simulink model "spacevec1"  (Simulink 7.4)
settings: Solver=ode45  StartTime=0.0  StopTime=.02  MaxStep=.00333  RelTol=1e-4
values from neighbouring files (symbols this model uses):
  j = sqrt(-1)    [im3d.m]    (also in imbar1.m; imbarB.m; imchplot66.m; imdef0vec.m)
libraries: simulink x2

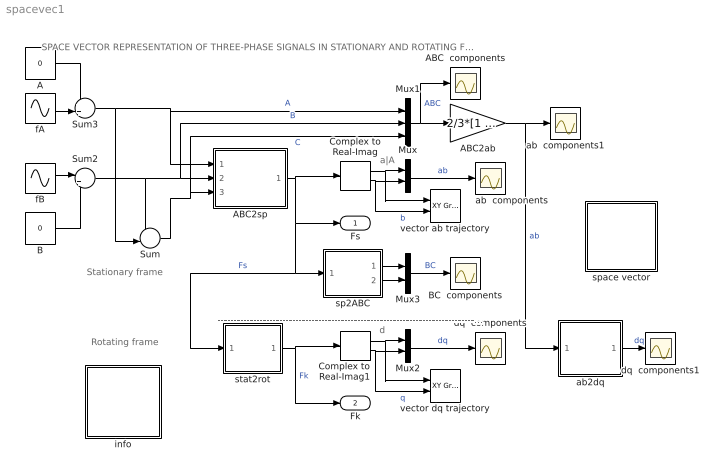
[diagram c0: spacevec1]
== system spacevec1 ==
  note: SPACE VECTOR REPRESENTATION OF THREE-PHASE SIGNALS IN STATIONARY AND ROTATING FRAMES
  note: a|A
  note: d
  note: Stationary frame
  note: ----------------------------------------------------------------------------------------------------------------------------------------------------------------------
  note: Rotating frame
  A : Constant  Value=0  OutDataType=sfix(16)  OutScaling=2^0
  ABC  components : Scope
  ABC2ab : Gain  Gain=2/3*[1 -0.5 -0.5;0 0.86667 -0.86667]  Multiplication=Matrix(K*u)  ParameterDataType=sfix(16)  ParameterScaling=2^0  OutDataType=sfix(16)  OutScaling=2^0
  ABC2sp : Subsystem
  B : Constant  Value=0  OutDataType=sfix(16)  OutScaling=2^0
  BC  components : Scope
  Complex to Real-Imag : ComplexToRealImag
  Complex to Real-Imag1 : ComplexToRealImag
  Mux : Mux  Inputs=2
  Mux1 : Mux  Inputs=3
  Mux2 : Mux  Inputs=2
  Mux3 : Mux  Inputs=2
  Sum : Sum  Inputs=--|  OutDataType=sfix(16)  OutScaling=2^0
  Sum2 : Sum  Inputs=|++  OutDataType=sfix(16)  OutScaling=2^0
  Sum3 : Sum  Inputs=++|  OutDataType=sfix(16)  OutScaling=2^0
  ab  components : Scope
  ab  components1 : Scope
  ab2dq : Subsystem
  dq  components : Scope
  dq  components1 : Scope
  fA : Sin  Amplitude=1  Bias=0  Frequency=2*pi*50  Phase=pi/2  Samples=10  SampleTime=0
  fB : Sin  Amplitude=1  Bias=0  Frequency=2*pi*50  Phase=-pi/6  Samples=10  SampleTime=0
  info : Subsystem
  sp2ABC : Subsystem
  space vector : Subsystem
  stat2rot : Subsystem
  vector ab trajectory : simulink/Sinks/XY Graph  SystemSampleTime=-1  xmin=-1  xmax=1  ymin=-1  ymax=1  st=-1
  vector dq trajectory : simulink/Sinks/XY Graph  SystemSampleTime=-1  xmin=-1  xmax=1  ymin=-1  ymax=1  st=-1
  Fs : Outport
  Fk : Outport  Port=2
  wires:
  Mux/1 -> ab  components/1  "ab"
  Complex to Real-Imag/1 -> Mux/1, vector ab trajectory/1
  Complex to Real-Imag/2 -> Mux/2, vector ab trajectory/2  "b"
  fB/1 -> Sum2/1
  B/1 -> Sum2/2
  Sum2/1 -> Sum/1, ABC2sp/2(B), Mux1/2  "B"
  Sum/1 -> ABC2sp/3(C), Mux1/3  "C"
  fA/1 -> Sum3/2
  A/1 -> Sum3/1
  Sum3/1 -> Sum/2, ABC2sp/1(A), Mux1/1  "A"
  Mux1/1 -> ABC2ab/1, ABC  components/1  "ABC"
  Mux2/1 -> dq  components/1  "dq"
  Complex to Real-Imag1/2 -> Mux2/2, vector dq trajectory/2  "q"
  Complex to Real-Imag1/1 -> Mux2/1, vector dq trajectory/1
  ABC2ab/1 -> ab  components1/1, ab2dq/1(ab)  "ab"
  ab2dq/1(dq) -> dq  components1/1  "dq"
  sp2ABC/1(B) -> Mux3/1
  sp2ABC/2(C) -> Mux3/2
  Mux3/1 -> BC  components/1  "BC"
  ABC2sp/1(sp) -> Complex to Real-Imag/1, Fs/1, sp2ABC/1(Fs), stat2rot/1(stat)  "Fs"
  stat2rot/1(rot) -> Complex to Real-Imag1/1, Fk/1  "Fk"

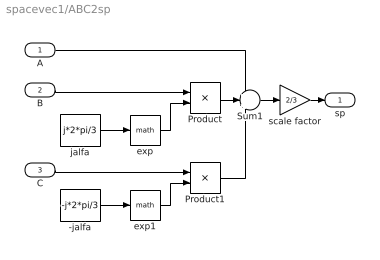
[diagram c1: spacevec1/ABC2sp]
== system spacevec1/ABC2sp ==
  A : Inport  OutDataType=sfix(16)  OutScaling=2^0
  B : Inport  Port=2  OutDataType=sfix(16)  OutScaling=2^0
  C : Inport  Port=3  OutDataType=sfix(16)  OutScaling=2^0
  -jalfa : Constant  Value=-j*2*pi/3  OutDataType=sfix(16)  OutScaling=2^0
  Product : Product  OutDataType=sfix(16)  OutScaling=2^0
  Product1 : Product  OutDataType=sfix(16)  OutScaling=2^0
  Sum1 : Sum  Inputs=+++  OutDataType=sfix(16)  OutScaling=2^0
  exp : Math
  exp1 : Math
  jalfa : Constant  Value=j*2*pi/3  OutDataType=sfix(16)  OutScaling=2^0
  scale factor : Gain  Gain=2/3  ParameterDataType=sfix(16)  ParameterScaling=2^0  OutDataType=sfix(16)  OutScaling=2^0
  sp : Outport
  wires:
  exp/1 -> Product/2
  jalfa/1 -> exp/1
  Product/1 -> Sum1/2
  exp1/1 -> Product1/2
  -jalfa/1 -> exp1/1
  Product1/1 -> Sum1/3
  B/1 -> Product/1
  C/1 -> Product1/1
  Sum1/1 -> scale factor/1
  scale factor/1 -> sp/1
  A/1 -> Sum1/1

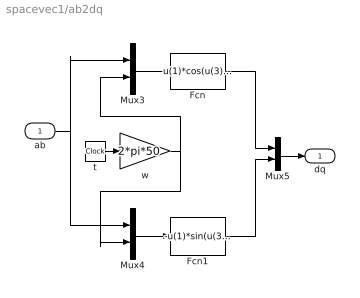
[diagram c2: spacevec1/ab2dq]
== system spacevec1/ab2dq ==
  ab : Inport  OutDataType=sfix(16)  OutScaling=2^0
  Fcn : Fcn  Expr=u(1)*cos(u(3))+u(2)*sin(u(3))
  Fcn1 : Fcn  Expr=-u(1)*sin(u(3))+u(2)*cos(u(3))
  Mux3 : Mux  Inputs=2
  Mux4 : Mux  Inputs=2
  Mux5 : Mux  Inputs=2
  t : Clock
  w : Gain  Gain=2*pi*50  ParameterDataType=sfix(16)  ParameterScaling=2^0  OutDataType=sfix(16)  OutScaling=2^0
  dq : Outport
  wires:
  t/1 -> w/1
  Mux3/1 -> Fcn/1
  Mux4/1 -> Fcn1/1
  w/1 -> Mux3/2, Mux4/2
  ab/1 -> Mux3/1, Mux4/1
  Fcn1/1 -> Mux5/2
  Fcn/1 -> Mux5/1
  Mux5/1 -> dq/1

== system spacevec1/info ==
  note: Space vector transformations
  note: This demonstration illustrates the use of a complex space vector to represent a three- phase signal . It also shows the transformation of the 3-phase signal 'ABC' into an equi- valent 2-phase system 'ab' . The only restriction to the 3-phase signal is that the zero- sequence component is zero i.e. fA+fB+fC=0. The complex space vector in the stationary frame is defined as Fs = 2/3 (fA + fB*exp(j2*pi/3) + fC*exp(-2j*pi/3) whose cartesian components are fa = Re (Fs) fb = Im (Fs) When expressed in a rotating frame at frequency wk, the space vector becomes Fk = Fs*exp(-jwk*t) whose cartesian components are fd = Re(Fk) fq = Im(Fk) The inverse transformation from complex space vector back to the 3-phase signal is also demonstrated. Finally, the real transformations of the ABC components to the components ab (in the stationary frame) and then dq (in the rotating frame) are shown.

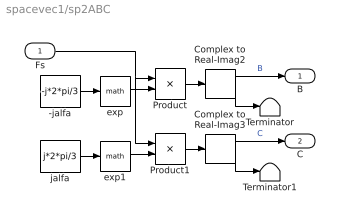
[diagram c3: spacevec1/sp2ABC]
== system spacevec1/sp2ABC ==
  Fs : Inport  OutDataType=sfix(16)  OutScaling=2^0
  -jalfa : Constant  Value=-j*2*pi/3  OutDataType=sfix(16)  OutScaling=2^0
  Complex to Real-Imag2 : ComplexToRealImag
  Complex to Real-Imag3 : ComplexToRealImag
  Product : Product  OutDataType=sfix(16)  OutScaling=2^0
  Product1 : Product  OutDataType=sfix(16)  OutScaling=2^0
  Terminator : Terminator
  Terminator1 : Terminator
  exp : Math
  exp1 : Math
  jalfa : Constant  Value=j*2*pi/3  OutDataType=sfix(16)  OutScaling=2^0
  B : Outport
  C : Outport  Port=2
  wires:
  exp/1 -> Product/2
  Product/1 -> Complex to Real-Imag2/1
  Complex to Real-Imag2/2 -> Terminator/1
  -jalfa/1 -> exp/1
  Complex to Real-Imag2/1 -> B/1  "B"
  Fs/1 -> Product/1, Product1/1
  exp1/1 -> Product1/2
  Product1/1 -> Complex to Real-Imag3/1
  Complex to Real-Imag3/2 -> Terminator1/1
  jalfa/1 -> exp1/1
  Complex to Real-Imag3/1 -> C/1  "C"

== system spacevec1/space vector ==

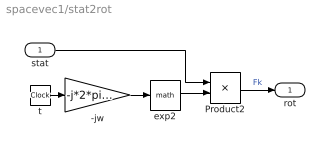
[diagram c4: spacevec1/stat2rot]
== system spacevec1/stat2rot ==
  stat : Inport  OutDataType=sfix(16)  OutScaling=2^0
  -jw : Gain  Gain=-j*2*pi*50  ParameterDataType=sfix(16)  ParameterScaling=2^0  OutDataType=sfix(16)  OutScaling=2^0
  Product2 : Product  OutDataType=sfix(16)  OutScaling=2^0
  exp2 : Math
  t : Clock
  rot : Outport
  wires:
  exp2/1 -> Product2/2
  -jw/1 -> exp2/1
  t/1 -> -jw/1
  Product2/1 -> rot/1  "Fk"
  stat/1 -> Product2/1
